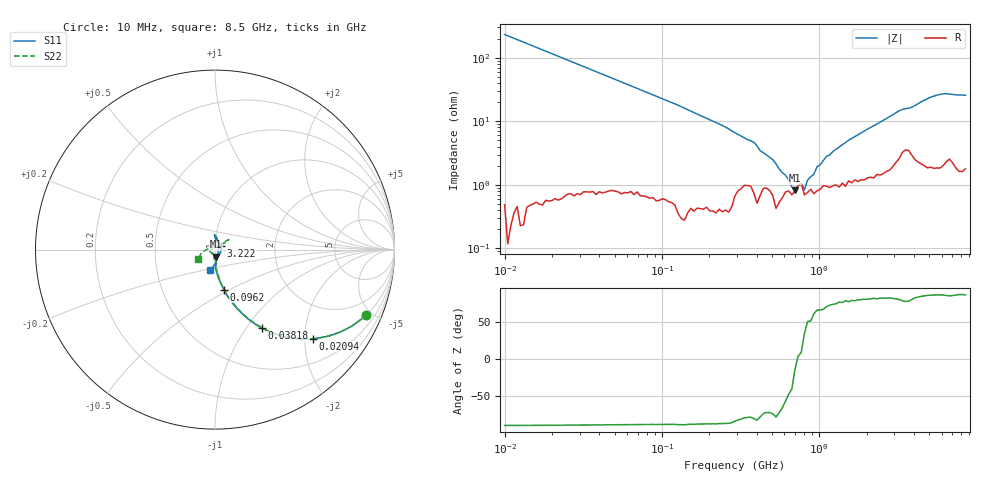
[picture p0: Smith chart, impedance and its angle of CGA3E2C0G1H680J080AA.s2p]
! S-parameter Generated by TDK Corporation
! Copyright(C) 2015 TDK Corporation.
! All Rights Reserved.
! TDK P/N: CGA3E2C0G1H680J080AA (Multilayer Ceramic Chip Capacitors)
! Property: C=68pF
! Size(LxWxT): 1.6x0.8x0.8mm, 0.063x0.031x0.031inches
! Model Type: s2p (Touchstone File Format Version 1.0)
! Frequency: DC=Yes Start=10MHz Stop=8500MHz 148points Log-sweep
! Note:
! Model Generated on Jun. 23, 2015
! Hash(MD5):
! Port Assignments:
!  1 ---| |--- 2
! Applicable Conditions:
!  Temperature = 25 degC
!  DC Bias Voltage = 0 V
!  Small Signal Operation
! Terms and conditions regarding TDK Simulation Models
! (1)This simulation model is being provided solely for informational purposes. Please refer to the specifications of the products in terms of detailed characteristics of such products.
! (2)In no event shall TDK Corporation of any of its subsidiaries be liable for any loss or damage arising, directly or indirectly,
!  From any information contained in this simulation model, including, but not limited to loss or damages arising from any inaccuracies, omissions or errors in connection with such information.
! (3)Any and all copyrights on this simulation model are owned by TDK Corporation.
!  Duplication or redistribution of this simulation model without prior written permission from TDK Corporation is prohibited.
! (4)This simulation model is subject to any modification or change without any prior notice.
! (5)Neither TDK Corporation nor any of its subsidiaries shall make any warranty, express or implied,
!  Including but not limited to the correctness, implied warranties of merchantability and fitness for a particular purpose with respect to this simulation models.
! (6)The use of this simulation model shall be deemed to have consented to the terms and conditions hereof.
# MHz S MA R 50
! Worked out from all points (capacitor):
!   147 points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, 10 MHz to 8.5 GHz, reference 50 ohm
!   read as one part in series: C = 68.6 pF near 10 MHz
!   lowest |Z| = 826 mohm at 701.4 MHz (marker M1)
!   series resonance near 727.3 MHz, so ESL is about 700 pH
!   S11 on the Smith chart (normalised r, x): 10 MHz: 1.01, -4.64; 20.94 MHz: 1.01, -2.19; 38.18 MHz: 1.01, -1.19; 96.2 MHz: 0.99, -0.47; 3.222 GHz: 1.07, +0.04; 8.5 GHz: 0.92, -0.21
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10  0.9173 -23.3  0.3951 66.6  0.3949 66.6  0.9172 -23.3
20.94268  0.7378 -42.2  0.6681 47.6  0.6684 47.6  0.7412 -42.0
31.74043  0.5826 -54.1  0.8033 35.7  0.8029 35.8  0.589 -53.5
38.18307  0.5108 -59.0  0.8492 30.8  0.8499 30.8  0.5194 -58.3
96.19692  0.2281 -77.7  0.961 13.0  0.9607 13.0  0.2407 -76.3
291.5476  0.08493 -86.0  0.9848 2.9  0.9824 2.9  0.07277 -88.1
507.5556  0.04368 -91.3  0.983 -0.0  0.9834 -0.1  0.05278 -94.0
701.3507  0.03913 -85.4  0.9844 -1.8  0.9832 -1.7  0.03078 -98.6
925.3847  0.0335 -74.7  0.9846 -3.2  0.9858 -3.2  0.03 -113.3
2226.117  0.03418 -28.6  0.9771 -10.5  0.9767 -10.3  0.02869 -163.7
2804.598  0.03237 3.3  0.9729 -13.2  0.9727 -13.2  0.01668 159.8
3076.094  0.03737 20.5  0.967 -14.6  0.9666 -14.5  0.01354 103.7
3221.545  0.03824 28.2  0.9637 -15.2  0.9622 -15.3  0.02006 70.4
3875.451  0.03916 56.9  0.9597 -17.2  0.9581 -17.0  0.03704 26.8
4451.596  0.06095 87.3  0.9652 -19.9  0.9651 -20.0  0.06859 35.5
5355.177  0.0853 92.2  0.9622 -24.3  0.9619 -24.3  0.09535 35.5
5873.579  0.07787 88.2  0.9596 -26.7  0.9584 -26.6  0.08616 36.7
6442.165  0.0485 69.8  0.9561 -29.1  0.9523 -29.0  0.06085 41.3
6746.777  0.02453 33.6  0.9524 -30.2  0.954 -30.1  0.03608 47.6
7065.792  0.02255 -40.1  0.9546 -31.3  0.9546 -31.2  0.01845 103.7
7749.789  0.07188 -86.9  0.9573 -34.6  0.9562 -34.3  0.06125 -172.5
8500  0.1192 -104.7  0.9535 -38.2  0.9523 -38.0  0.1067 -149.7
